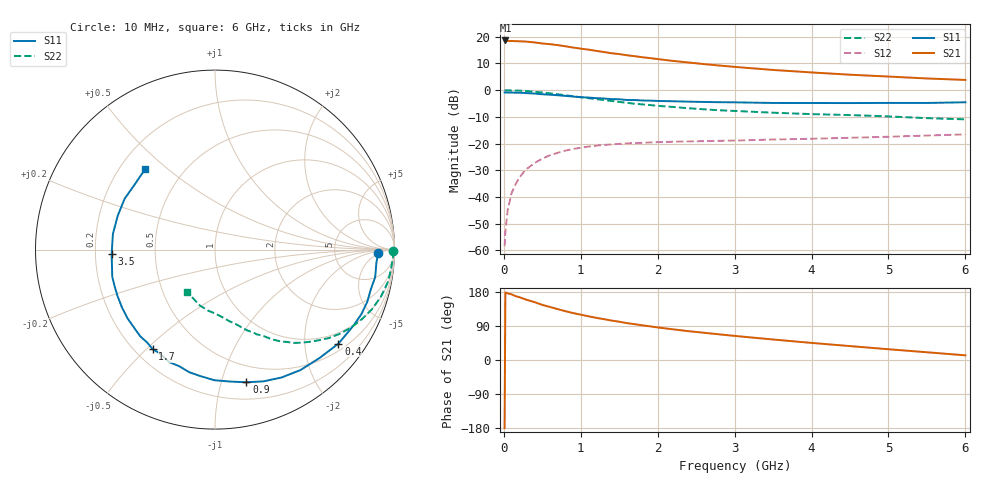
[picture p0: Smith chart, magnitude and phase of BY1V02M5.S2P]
! SIEMENS Small Signal Semiconductors
! BFY420
! Si NPN RF SIEGET Grounded Emitter Transistor in MICRO-X
! VCE = 1 V  IC = 2.5 mA
! Common Emitter S-Parameters:  October  1996
# GHz  S  MA  R  50
!  f  S11  S21  S12  S22
! GHz  MAG  ANG  MAG  ANG  MAG  ANG  MAG  ANG
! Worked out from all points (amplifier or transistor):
!   36 points, 10 MHz to 6 GHz, reference 50 ohm
!   highest |S21| = 18.6 dB at 20 MHz (marker M1)
!   |S21| within 3 dB of that: start of sweep to 983.3 MHz
!   unconditionally stable (mu >= 1): 3.754 GHz to end of sweep
!   at 250 MHz: K = 0.06, MSG = 24.6 dB, |S12| = -30.9 dB
!   at 1.4 GHz: K = 0.36, MSG = 17.1 dB, |S12| = -20.3 dB
!   at 6 GHz: K = 1.24, MAG = 7.3 dB, |S12| = -16.6 dB
!   S11 on the Smith chart (normalised r, x): 10 MHz: 19, -4; 400 MHz: 0.68, -2.82; 900 MHz: 0.34, -1.20; 1.7 GHz: 0.27, -0.52; 3.5 GHz: 0.27, -0.02; 6 GHz: 0.30, +0.42
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0.01  0.9063 -1.2  8.474 -179.7  0.0012 104.1  0.9945 -0.5
0.02  0.9066 -2.1  8.534 178.2  0.0022 89.3  0.9918 -1.0
0.05  0.9023 -4.7  8.339 175.9  0.0057 87.1  0.9924 -2.7
0.1  0.9055 -9.8  8.334 173.3  0.0117 85.5  0.9875 -5.4
0.15  0.8959 -14.3  8.293 168.7  0.0171 81.3  0.9839 -8.1
0.3  0.8811 -28.4  8.098 158.6  0.0338 73.5  0.9601 -16.0
0.4  0.8646 -37.3  7.84 152.7  0.0434 68.2  0.9346 -21.0
0.5  0.8391 -46.0  7.494 145.4  0.0523 63.9  0.9046 -25.5
0.6  0.823 -54.6  7.273 139.9  0.0605 59.5  0.8728 -29.9
0.7  0.8036 -62.4  6.984 134.3  0.0672 55.4  0.8378 -34.1
0.8  0.7822 -69.8  6.638 128.8  0.0737 50.8  0.8036 -37.8
0.9  0.7597 -76.7  6.285 123.9  0.0794 47.6  0.7692 -41.0
1.1  0.7277 -90.3  5.748 115.3  0.0879 41.9  0.7079 -47.1
1.4  0.6795 -107.1  4.917 104.1  0.0963 34.6  0.6294 -54.4
1.7  0.6539 -122.1  4.333 94.5  0.1021 29.5  0.5569 -60.3
2  0.6286 -134.8  3.824 85.9  0.1062 25.4  0.5095 -65.1
2.2  0.62 -141.7  3.532 80.9  0.1084 23.1  0.4852 -68.2
2.8  0.5956 -159.8  2.896 67.7  0.1128 18.8  0.4209 -75.9
3.5  0.5764 -177.5  2.393 54.1  0.1193 15.9  0.3788 -83.8
4.5  0.5739 160.8  1.949 36.7  0.1284 12.2  0.3423 -96.4
5.5  0.5766 140.2  1.657 20.4  0.1415 9.1  0.2994 -113.4
6  0.5939 131.0  1.556 12.3  0.1487 7.2  0.2845 -123.5
